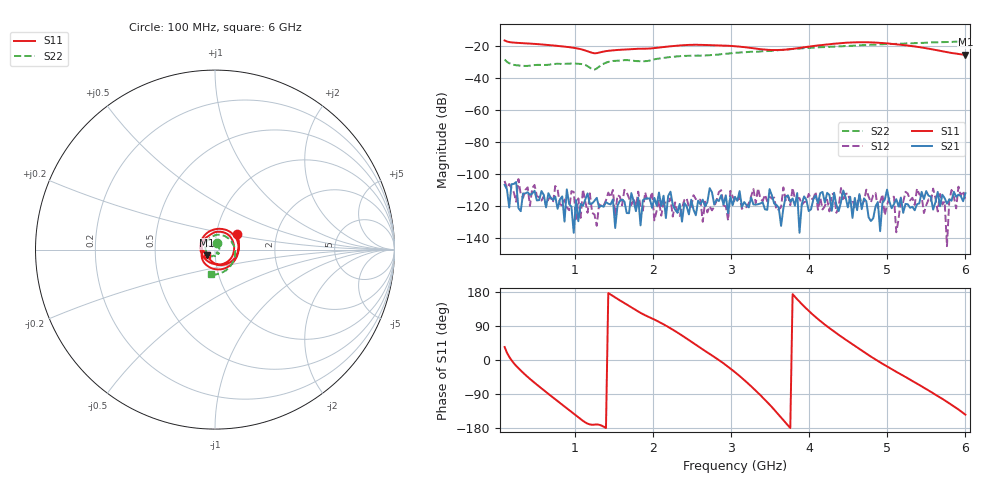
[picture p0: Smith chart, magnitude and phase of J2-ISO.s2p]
!Agilent Technologies,E8364B,MY43040379,A.07.50.67
!Agilent E8364B: A.07.50.67
!Date: Tuesday, March 24, 2026 10:36:20
!Correction: S11(Full 2 Port(1,2))
!S21(Full 2 Port(1,2))
!S12(Full 2 Port(1,2))
!S22(Full 2 Port(1,2))
!S2P File: Measurements: S11, S21, S12, S22:
# Hz S  dB  R 50
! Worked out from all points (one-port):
!   201 points, 100 MHz to 6 GHz, reference 50 ohm
!   lowest |S11| = -25.3 dB at 6 GHz (marker M1), VSWR 1.11, Z = 45.7 - j2.91 ohm
!   |S11| at or under -10 dB: start of sweep to end of sweep
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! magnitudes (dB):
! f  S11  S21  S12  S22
! 100 MHz  -16.4  -106.6  -104.2  -28.3
! 129.5 MHz  -17.0  -109.3  -108.7  -29.7
! 188.5 MHz  -17.6  -106.2  -108.8  -31.2
! 336 MHz  -18.1  -112.0  -114.8  -32.2
! 778.5 MHz  -19.8  -121.6  -109.5  -30.9
! 1.103 GHz  -22.2  -119.7  -109.4  -31.3
! 1.25 GHz  -24.4  -116.6  -125.2  -34.6
! 1.369 GHz  -23.3  -120.3  -119.7  -30.9
! 1.457 GHz  -22.7  -118.9  -114.3  -29.4
! 1.663 GHz  -22.0  -124.2  -111.3  -28.7
! 1.899 GHz  -21.5  -115.3  -111.3  -29.4
! 2.076 GHz  -20.8  -111.4  -116.3  -27.7
! 2.49 GHz  -19.1  -115.9  -120.3  -26.0
! 2.814 GHz  -19.4  -115.8  -116.4  -25.3
! 3.05 GHz  -20.0  -114.1  -116.8  -24.1
! 3.551 GHz  -22.4  -118.3  -114.5  -22.7
! 3.728 GHz  -22.0  -113.2  -113.3  -22.0
! 4.053 GHz  -19.9  -115.7  -115.2  -20.9
! 4.614 GHz  -17.5  -122.4  -118.9  -19.5
! 5.027 GHz  -18.3  -116.9  -115.0  -18.6
! 5.38 GHz  -20.3  -118.7  -108.9  -18.0
! 6 GHz  -25.3  -111.9  -116.0  -17.1
